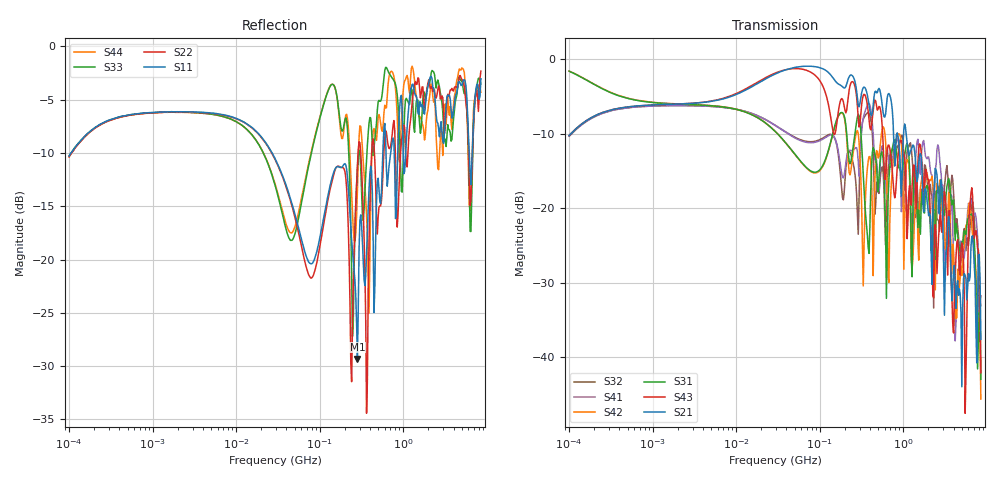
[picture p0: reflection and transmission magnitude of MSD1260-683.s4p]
# MHz S MA R 50
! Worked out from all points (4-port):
!   498 points, 100 kHz to 8.5 GHz, reference 50 ohm
!   strongest paths, dB at 100 kHz, 1.698 MHz, 29.49 MHz, 500.7 MHz, 8.5 GHz:
!     S21: -10.2, -6.0, -2.0, -4.1, -37.6
!     S43: -10.2, -6.0, -1.8, -6.7, -42.1
!     S31: -1.6, -6.0, -9.7, -17.8, -43.0
!     S42: -1.6, -6.0, -9.7, -13.3, -45.6
!     S41: -10.3, -6.2, -8.9, -17.8, -33.1
!     S32: -10.3, -6.2, -8.9, -17.8, -31.8
!   lowest |S11| = -29.3 dB at 282.9 MHz (marker M1), VSWR 1.07, Z = 53.3 - j1.25 ohm
!   |S11| at or under -10 dB: 26.97 MHz to 570 MHz (543 MHz wide, 182 % of centre); 621.9 MHz to 706.7 MHz (84.84 MHz wide, 12.8 % of centre); 6.173 GHz to 6.683 GHz (510.5 MHz wide, 7.94 % of centre)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
0.1  0.3058 50.1  0.3082 50.6  0.8322 -16.6  0.3048 -130.0
     0.3082 50.6  0.3031 50.0  0.3045 -130.0  0.8333 -16.6
     0.8322 -16.6  0.3045 -130.0  0.3063 50.1  0.3077 50.6
     0.3048 -130.0  0.8333 -16.6  0.3077 50.6  0.3043 50.1
282.8688  0.0341 -20.1  0.5491 -69.8  0.4102 -13.0  0.2411 19.3
          0.5491 -69.8  0.2775 24.2  0.08915 0.9  0.3324 -21.5
          0.4102 -13.0  0.08915 0.9  0.2667 6.3  0.4826 -82.2
          0.2411 19.3  0.3324 -21.5  0.4826 -82.2  0.2119 4.2
2209.207  0.7071 172.4  0.03085 -92.1  0.0566 147.2  0.1676 112.4
          0.03085 -92.1  0.648 177.1  0.1195 99.6  0.1642 111.2
          0.0566 147.2  0.1195 99.6  0.7714 177.4  0.05684 77.2
          0.1676 112.4  0.1642 111.2  0.05684 77.2  0.641 169.0
3488.216  0.5877 16.5  0.08792 -156.9  0.1585 5.9  0.106 -5.6
          0.08792 -156.9  0.583 12.9  0.1446 1.8  0.1273 -1.2
          0.1585 5.9  0.1446 1.8  0.4075 -0.9  0.08144 39.1
          0.106 -5.6  0.1273 -1.2  0.08144 39.1  0.5037 6.9
4913.36  0.6557 -95.5  0.0198 58.8  0.05516 -123.6  0.06038 -98.7
         0.0198 58.8  0.7135 -100.1  0.04452 -117.4  0.0407 -101.8
         0.05516 -123.6  0.04452 -117.4  0.6892 -93.0  0.05252 -171.4
         0.06038 -98.7  0.0407 -101.8  0.05252 -171.4  0.7753 -93.8
6462.473  0.2246 111.7  0.0547 48.7  0.09095 55.0  0.117 98.9
          0.0547 48.7  0.1915 71.9  0.09069 95.9  0.09256 53.4
          0.09095 55.0  0.09069 95.9  0.1354 90.5  0.1265 63.9
          0.117 98.9  0.09256 53.4  0.1265 63.9  0.207 46.5
8500  0.7048 -37.2  0.01318 -145.3  0.007109 165.5  0.02219 -139.1
      0.01318 -145.3  0.7656 -45.0  0.02583 -169.8  0.00524 -131.7
      0.007109 165.5  0.02583 -169.8  0.6659 -50.3  0.007868 148.2
      0.02219 -139.1  0.00524 -131.7  0.007868 148.2  0.6102 -58.6
